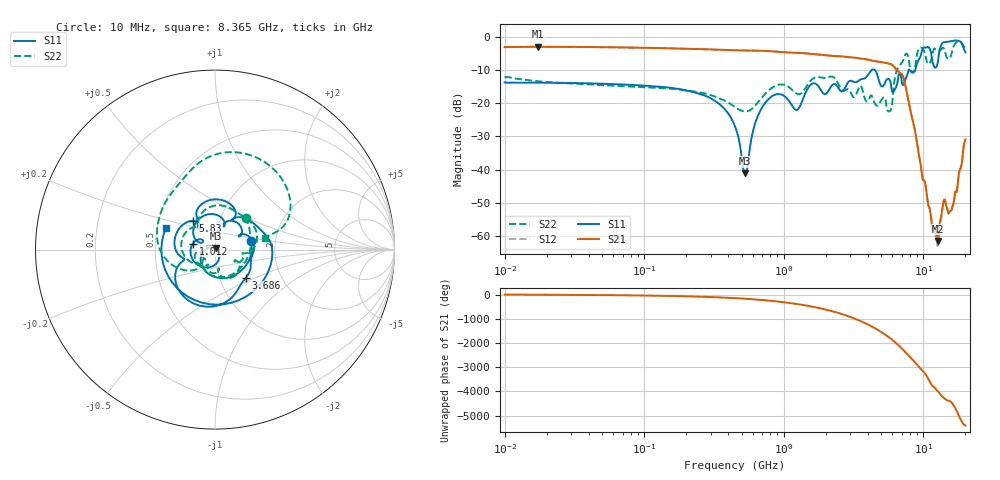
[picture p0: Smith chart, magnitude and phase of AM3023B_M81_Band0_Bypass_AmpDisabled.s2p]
!Agilent Technologies,E8364B,MY43040894,A.07.50.67
!Agilent E8364B: A.07.50.67
!Date: Tuesday, October 27, 2020 10:39:56
!Correction: S11(Full 2 Port(1,2))
!S21(Full 2 Port(1,2))
!S12(Full 2 Port(1,2))
!S22(Full 2 Port(1,2))
!S2P File: Measurements: S11, S21, S12, S22:Log Frequency Sweep
# Hz S  dB  R 50
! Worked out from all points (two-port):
!   3201 points, 10 MHz to 20 GHz, reference 50 ohm
!   highest |S21| = -2.98 dB at 17.39 MHz (marker M1); lowest = -61.5 dB at 12.65 GHz (marker M2)
!   |S21| within 3 dB of the highest: start of sweep to 2.754 GHz
!   lowest |S11| = -41.1 dB at 529.4 MHz (marker M3), VSWR 1.02, Z = 50.5 + j0.759 ohm
!   |S11| at or under -10 dB: start of sweep to 4.269 GHz; 4.494 GHz to 7.825 GHz (3.332 GHz wide, 54.1 % of centre); 7.961 GHz to 8.75 GHz (789.2 MHz wide, 9.45 % of centre)
!   |S22| runs from -22.5 to -1.4 dB; largest |S21 - S12| = 0.0064
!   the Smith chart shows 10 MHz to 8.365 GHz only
!   S11 on the Smith chart (normalised r, x): 10 MHz: 1.49, +0.14; 1.012 GHz: 0.78, +0.05; 3.686 GHz: 1.33, -0.45; 5.83 GHz: 0.75, +0.25; 8.365 GHz: 0.56, +0.15
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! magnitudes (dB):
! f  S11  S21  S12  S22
! 10 MHz  -13.7  -3.1  -3.0  -12.2
! 17.39 MHz  -13.8  -3.0  -3.0  -13.4
! 35.55 MHz  -14.0  -3.0  -3.1  -14.2
! 126.1 MHz  -15.0  -3.3  -3.4  -15.4
! 295.1 MHz  -18.4  -3.8  -3.8  -17.4
! 447.2 MHz  -27.0  -4.0  -4.1  -21.2
! 529.4 MHz  -41.1  -4.1  -4.1  -22.4
! 682.6 MHz  -22.1  -4.2  -4.2  -18.7
! 1.012 GHz  -17.9  -4.6  -4.6  -14.5
! 1.245 GHz  -22.0  -4.8  -4.8  -17.1
! 1.59 GHz  -14.2  -5.1  -5.2  -12.8
! 3.686 GHz  -12.6  -6.6  -6.7  -16.4
! 5.639 GHz  -12.7  -8.0  -8.0  -22.5
! 5.83 GHz  -13.9  -8.2  -8.2  -22.1
! 6.396 GHz  -14.9  -9.9  -9.8  -10.6
! 7.358 GHz  -13.4  -13.9  -13.7  -5.7
! 8.365 GHz  -10.5  -24.9  -25.0  -10.8
! 10.28 GHz  -3.2  -43.8  -44.1  -5.1
! 12.65 GHz  -8.0  -61.5  -63.0  -4.1
! 14.04 GHz  -1.6  -49.2  -49.4  -3.6
! 16.11 GHz  -1.2  -51.3  -51.1  -4.1
! 20 GHz  -4.7  -30.9  -31.3  -3.5
